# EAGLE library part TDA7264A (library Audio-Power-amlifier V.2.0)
The TDA7264A is class AB dual Audio power amplifier assembled in the Multiwatt package, specially designed for high quality sound application as Hi-Fi music centers and stereo TV sets.
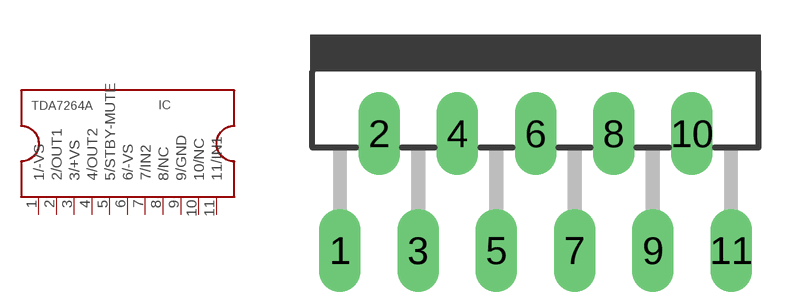
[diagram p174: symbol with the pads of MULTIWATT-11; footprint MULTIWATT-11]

Designator prefix IC

## TDA7264A  [MULTIWATT-11]
1  1/-VS  pwr
2  2/OUT1  out
3  3/+VS  pwr
4  4/OUT2  out
5  5/STBY-MUTE  in
6  6/-VS  pwr
7  7/IN2  in
8  8/NC  nc
9  9/GND  pwr
10  10/NC  nc
11  11/IN1  in

## Footprint MULTIWATT-11 (pad centres in mm)
Muliwatt 11 lead
drill 1.2 long: 1 -8.5,-6.35; 2 -6.8,-1.27; 3 -5.1,-6.35; 4 -3.4,-1.27; 5 -1.7,-6.35; 6 0,-1.27; 7 1.7,-6.35; 8 3.4,-1.27; 9 5.1,-6.35; 10 6.8,-1.27; 11 8.5,-6.35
